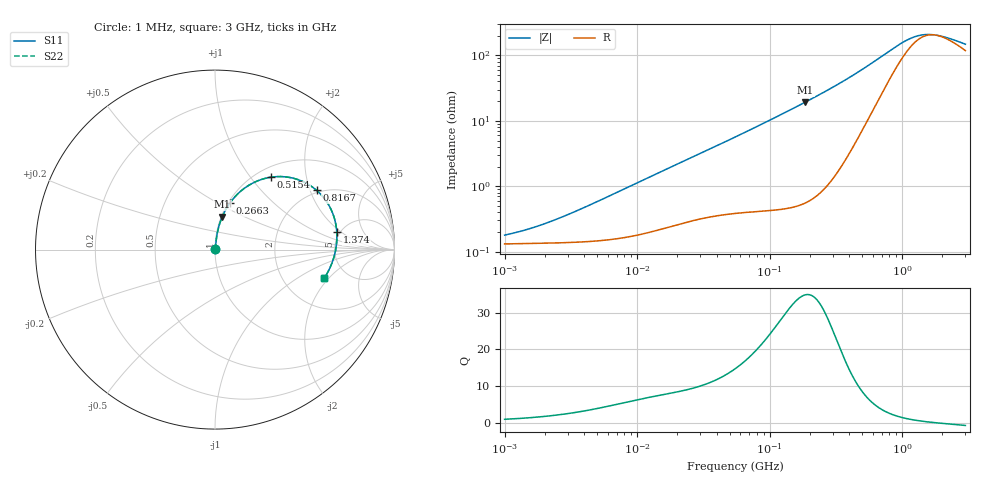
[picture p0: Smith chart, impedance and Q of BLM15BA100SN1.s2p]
! BLM15BA100SN1
# Hz S RI R 50
!Freq.(Hz) S11(Real) S11(Imag) S21(Real) S21(Imag) S12(Real) S12(Imag) S22(Real) S22(Imag)
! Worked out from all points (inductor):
!   401 points, 1 MHz to 3 GHz, reference 50 ohm
!   read as one part in series: L = 18 nH near 3.747 MHz
!   highest Q = 34.8 at 185.7 MHz (marker M1), where L = 16.5 nH
!   self-resonance near 1.776 GHz
!   S11 on the Smith chart (normalised r, x): 1 MHz: 1.00, +0.00; 266.3 MHz: 1.02, +0.57; 515.4 MHz: 1.16, +1.26; 816.7 MHz: 1.92, +2.22; 1.374 GHz: 4.69, +1.73; 3 GHz: 3.37, -1.78
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1000000  0.00131 0.00121  0.9987 -0.00121  0.9987 -0.00121  0.00131 0.00121
1350181  0.00133 0.00159  0.9987 -0.00159  0.9987 -0.00159  0.00133 0.00159
1859846  0.00134 0.00214  0.9987 -0.00214  0.9987 -0.00214  0.00134 0.00214
3823119  0.00142 0.00432  0.9986 -0.00432  0.9986 -0.00432  0.00142 0.00432
1.461624e7  0.0024 0.0159  0.9976 -0.0159  0.9976 -0.0159  0.0024 0.0159
5.477226e7  0.00693 0.0556  0.9931 -0.0556  0.9931 -0.0556  0.00693 0.0556
1.060286e8  0.0157 0.106  0.9843 -0.106  0.9843 -0.106  0.0157 0.106
1.857042e8  0.0408 0.184  0.9592 -0.184  0.9592 -0.184  0.0408 0.184
2.094008e8  0.0513 0.2067  0.9487 -0.2067  0.9487 -0.2067  0.0513 0.2067
2.662515e8  0.0829 0.2592  0.9171 -0.2592  0.9171 -0.2592  0.0829 0.2592
3.741707e8  0.1668 0.344  0.8332 -0.344  0.8332 -0.344  0.1668 0.344
4.391493e8  0.23 0.3799  0.77 -0.3799  0.77 -0.3799  0.23 0.3799
5.154121e8  0.3102 0.4031  0.6898 -0.4031  0.6898 -0.4031  0.3102 0.4031
6.423554e8  0.438 0.3972  0.562 -0.3972  0.562 -0.3972  0.438 0.3972
8.005644e8  0.557 0.3379  0.443 -0.3379  0.443 -0.3379  0.557 0.3379
8.167498e8  0.5661 0.3303  0.4339 -0.3303  0.4339 -0.3303  0.5661 0.3303
1.038491e9  0.6464 0.224  0.3536 -0.224  0.3536 -0.224  0.6464 0.224
1.194682e9  0.6692 0.1591  0.3308 -0.1591  0.3308 -0.1591  0.6692 0.1591
1.374365e9  0.6784 0.098  0.3216 -0.098  0.3216 -0.098  0.6784 0.098
1.581072e9  0.678 0.0423  0.322 -0.0423  0.322 -0.0423  0.678 0.0423
1.855641e9  0.6694 -0.0152  0.3306 0.0152  0.3306 0.0152  0.6694 -0.0152
3e9  0.608 -0.16  0.392 0.16  0.392 0.16  0.608 -0.16
